(* Logix 5000 AddOnInstructionDefinition export AMP_Alarm_Reset; software revision 20.04 *)

TYPE AMP_Status_Word :   // Applied Motion Input Assembly Status Word
STRUCT
   Enabled : BOOL;   // Motor Enabled (Motor Disabled if this bit = 0)
   Sampling : BOOL;   // Sampling (for Quick Tuner)
   Drive_Fault : BOOL;   // Drive Fault (check Alarm Code)
   In_Position : BOOL;   // In Position (motor is in position)
   Moving : BOOL;   // Moving (motor is moving)
   Jogging : BOOL;   // Jogging (currently in jog mode)
   Stopping : BOOL;   // Stopping (in the process of stopping from a stop command)
   Waiting : BOOL;   // Waiting (for an input; executing a WI command)
   Saving : BOOL;   // Saving (parameter data is being saved)
   Alarm_Present : BOOL;   // Alarm present (check Alarm Code)
   Homing : BOOL;   // Homing (executing an SH command)
   Wait_Time : BOOL;   // Waiting (for time; executing a WD or WT command)
   Wizard_Running : BOOL;   // Wizard running (Timing Wizard is running)
   Checking_Encoder : BOOL;   // Checking encoder (Timing Wizard is running)
   Q_Program_Running : BOOL;   // Q Program is running
   Initializing : BOOL;   // Initializing (happens at power up) ; Servo Ready (for SV200 drives only)
END_STRUCT
END_TYPE

TYPE AMP_Input_Assembly_v2 :   // Applied Motion Drive Input Assembly Version 2.0
STRUCT
   Status_Code : DINT;   // Status Code
   Alarm_Code : DINT;   // Alarm Code
   Voltage : DINT;   // Supply Voltage (x0.1V)
   Current : DINT;   // Actual Current (mA)
   Temp : DINT;   // Drive Temperature (0.1 deg C)
   Encoder_Position : DINT;   // Encoder Position (20,000 counts = 1 shaft turn)
   Absolute_Position : DINT;   // Absolute Position (20,000 counts = 1 shaft turn)
   Position_Error : DINT;   // Position Error (counts)
   Actual_Velocity : DINT;   // Actual Velocity (rev/sec * 240, 0 when no encoder)
   Extended_Inputs : DINT;   // Input Status (Extended)
   Main_Board_Inputs : DINT;   // Input Status (Main board)
   Word11 : DINT;   // Reserved
   Analog_Input_1 : DINT;   // Analog Input 1 (ADC counts, 0=min V, 16383 = max V)
   Analog_Input_2 : DINT;   // Analog Input 2 (ADC counts, 0=min V, 16383 = max V)
END_STRUCT
END_TYPE

ADD_ON_INSTRUCTION AMP_Alarm_Reset   (* revision 1.0 *)
// Applied Motion - Alarm Reset - AOI
// Help:
// The Alarm Reset AOI is used to reset Drive Fault and clear Alarm Code (if possible). Figure 1 shows a preview of an instance of the AOI.
VAR_IN_OUT
   Input : DINT[14]; {required}   // Drive Input Assembly
   Output : DINT[16]; {required}   // Drive Output Assembly
        [0]   // Command Word
        [1]   // Jog Speed (0.25 rev/min)
        [2]   // Jog Acceleration (10 rev/s/s)
        [3]   // Jog Deceleration (10 rev/s/s)
        [4]   // Point-to-Point Velocity (0.25 rev/min)
        [5]   // Point-to-Point Acceleration (10 rev/s/s)
        [6]   // Point-to-Point Deceleration (10 rev/s/s)
        [7]   // Point-to-Point Distance (Motor steps)
        [9]   // (2x ASCII Letters in 16 lower word)
        [10]   // Data/Register 1
        [11]   // Data/Register 2
END_VAR
VAR_INPUT
   RPI : DINT := 100; {visible}   // Drive Connection Request Packet Interval (milliseconds)
   Reset : BOOL; {required}   // Reset the Drive (on rising edge)
END_VAR
VAR_OUTPUT
   Sent : BOOL; {access Read Only, visible}   // Reset has been sent to drive
   In_Progress : BOOL; {access Read Only, visible}   // Reset in progress
   Done : BOOL; {access Read Only, visible}   // Reset completed without errors - Drive is not faulted
   Error : BOOL; {access Read Only, visible}   // Reset failed - Not Used
   State : DINT := 10; {access None}   // Internal state of progress
END_VAR
VAR
   Loc_StatusCode : AMP_Status_Word;
   Loc_CommandOff_Timer : TIMER;   // Timer to make sure command value was 0 before sending a new command
   Loc_CommandOn_Timer : TIMER;   // Timer to make sure command value is set long enough to be sent to servo
   Loc_Input_Assembly : AMP_Input_Assembly_v2; {access None}
   Loc_Stop_ONS : BOOL; {access None}
END_VAR

ROUTINE Logic   (* ladder *)
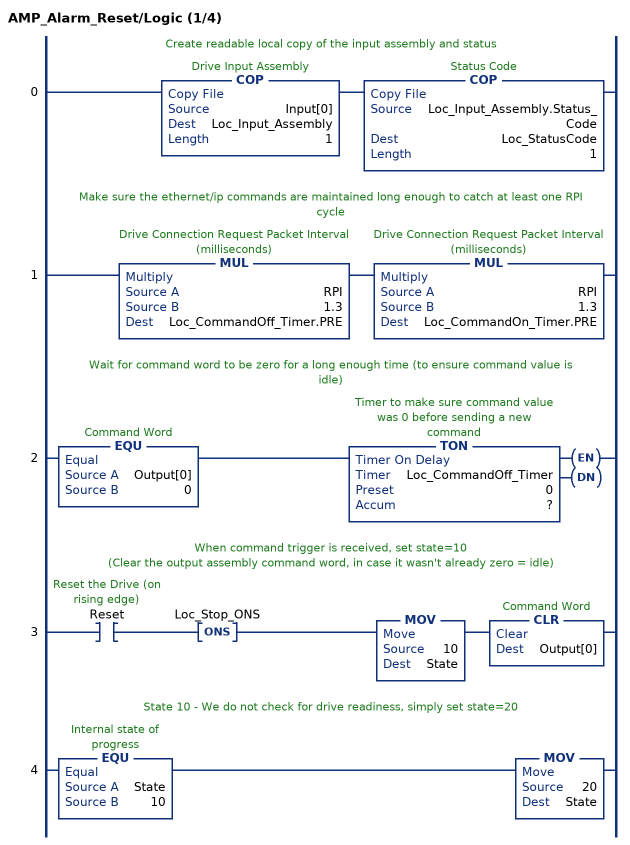
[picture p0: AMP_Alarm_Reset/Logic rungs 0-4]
   // Create readable local copy of the input assembly and status
   0: COP(Input[0],Loc_Input_Assembly,1)COP(Loc_Input_Assembly.Status_Code,Loc_StatusCode,1);
   // Make sure the ethernet/ip commands are maintained long enough to catch at least one RPI cycle
   1: MUL(RPI,1.3,Loc_CommandOff_Timer.PRE)MUL(RPI,1.3,Loc_CommandOn_Timer.PRE);
   // Wait for command word to be zero for a long enough time (to ensure command value is idle)
   2: EQU(Output[0],0)TON(Loc_CommandOff_Timer,?,?);
   // When command trigger is received, set state=10
   // (Clear the output assembly command word, in case it wasn't already zero = idle)
   3: XIC(Reset)ONS(Loc_Stop_ONS)MOV(10,State)CLR(Output[0]);
   // State 10 - We do not check for drive readiness, simply set state=20
   4: EQU(State,10)MOV(20,State);
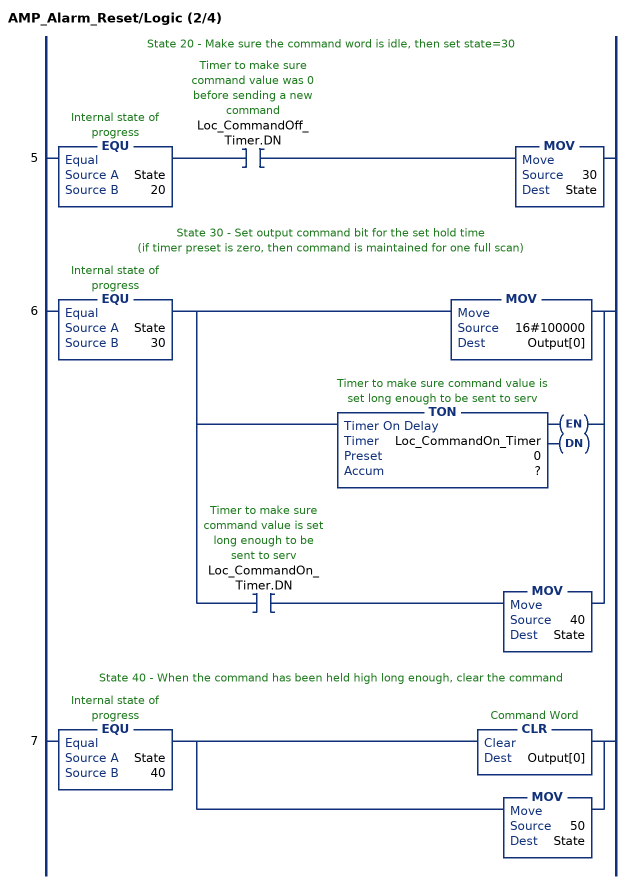
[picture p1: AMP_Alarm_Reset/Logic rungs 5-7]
   // State 20 - Make sure the command word is idle, then set state=30
   5: EQU(State,20)XIC(Loc_CommandOff_Timer.DN)MOV(30,State);
   // State 30 - Set output command bit for the set hold time
   // (if timer preset is zero, then command is maintained for one full scan)
   6: EQU(State,30)[MOV(16#100000,Output[0]) ,TON(Loc_CommandOn_Timer,?,?) ,XIC(Loc_CommandOn_Timer.DN) MOV(40,State) ];
   // State 40 - When the command has been held high long enough, clear the command
   7: EQU(State,40)[CLR(Output[0]) ,MOV(50,State) ];
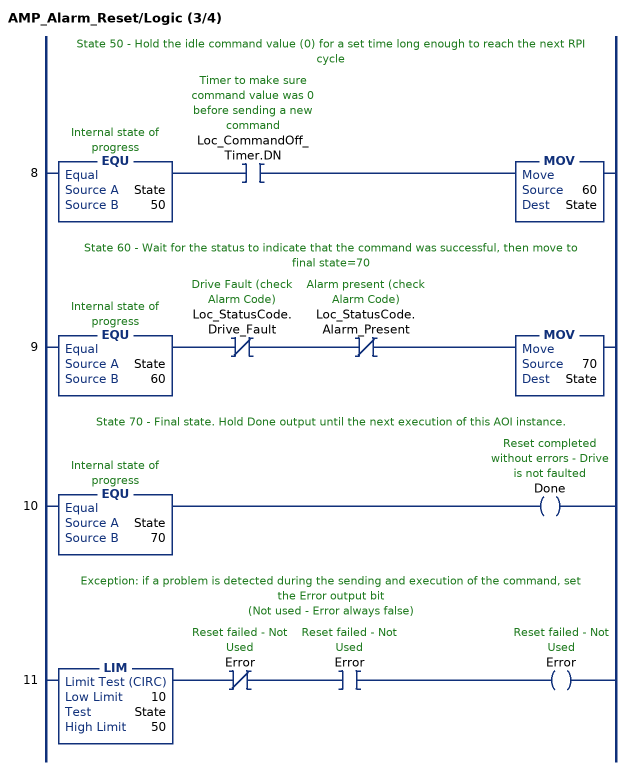
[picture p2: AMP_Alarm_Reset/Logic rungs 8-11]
   // State 50 - Hold the idle command value (0) for a set time long enough to reach the next RPI cycle
   8: EQU(State,50)XIC(Loc_CommandOff_Timer.DN)MOV(60,State);
   // State 60 - Wait for the status to indicate that the command was successful, then move to final state=70
   9: EQU(State,60)XIO(Loc_StatusCode.Drive_Fault)XIO(Loc_StatusCode.Alarm_Present)MOV(70,State);
   // State 70 - Final state. Hold Done output until the next execution of this AOI instance.
   10: EQU(State,70)OTE(Done);
   // Exception: if a problem is detected during the sending and execution of the command, set the Error output bit
   // (Not used - Error always false)
   11: LIM(10,State,50)XIO(Error)XIC(Error)OTE(Error);
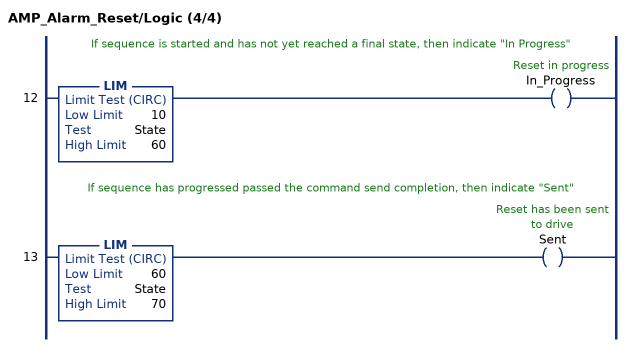
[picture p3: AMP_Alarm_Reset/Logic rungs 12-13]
   // If sequence is started and has not yet reached a final state, then indicate "In Progress"
   12: LIM(10,State,60)OTE(In_Progress);
   // If sequence has progressed passed the command send completion, then indicate "Sent"
   13: LIM(60,State,70)OTE(Sent);
END_ROUTINE
END_ADD_ON_INSTRUCTION
